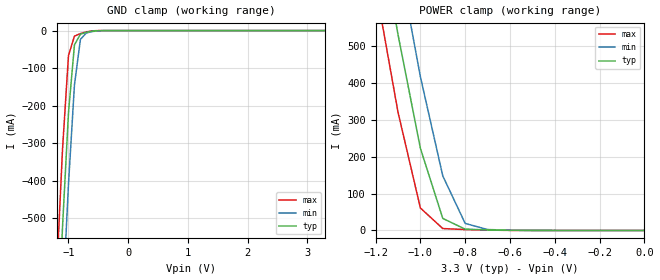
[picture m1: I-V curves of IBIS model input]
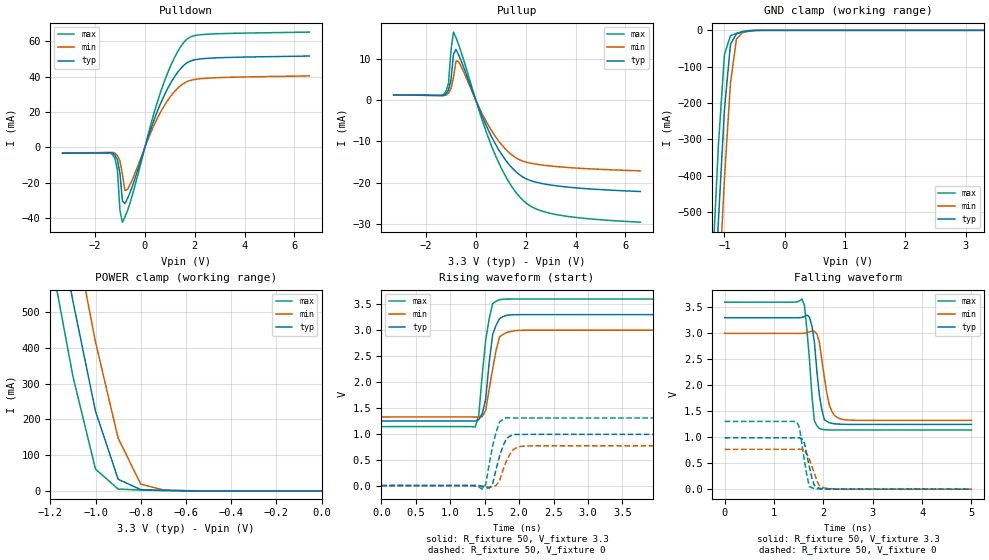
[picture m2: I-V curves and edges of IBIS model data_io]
| TSOP package & Industrial   Operation
[IBIS Ver]   3.2
[Comment Char]   |_char
[File name]   as7c31026b_tsopi.ibs
[File Rev]   1.0
[Date]   May 19, 2004 3:37:27 PM
[Source]
Alliance Semiconductor Corporation
[Notes]
This model  is for TSOP package &
 Industrial  Operation
[Disclaimer]
Data is for modeling purpose only and is not guaranted.
This IBIS model is provided on an "AS IS" basis and Alliance Semiconductor makes
absolutely no warranty with respect to the information contained
herein.The entire risk as to quality and performance
is with the Customer. ACCORDINGLY, IN NO EVENT SHALL THE COMPANY BE
LIABLE FOR ANY DAMAGES, WHETHER IN CONTRACT OR TORT,INCLUDING ANY
LOST PROFITS OR OTHER INCIDENTAL, CONSEQUENTIAL, EXEMPLARY, OR
PUNITIVE DAMAGES ARISING OUT OF THE USE OR APPLICATION OF THE IBIS
model provided in this package.
[Copyright]
Alliance Semiconductor Corporation
| tsop Package & Industrial Operation.
[Component]   AS7C31026B_TSOPI
Si_location Pin
Timing_location Pin
[Manufacturer]   Alliance Semiconductor Corporation
[Package]
R_pkg   321.15m   142.5m   499.8m
L_pkg   5.882nH   2.534nH   9.23nH
C_pkg   1.013pF   0.614pF   1.412pF
[Pin] signal_name   model_name
1   A4   input
2   A3   input
3   A2   input
4   A1   input
5   A0   input
6   NCE   input
7   IO0   data_io
8   IO1   data_io
9   IO2   data_io
10   IO3   data_io
11   VCC   POWER
12   GND   GND
13   IO4   data_io
14   IO5   data_io
15   IO6   data_io
16   IO7   data_io
17   NWE   input
18   A15   input
19   A14   input
20   A13   input
21   A12   input
22   NC   NC
23   NC   NC
24   A11   input
25   A10   input
26   A9   input
27   A8   input
28   NC   NC
29   IO8   data_io
30   IO9   data_io
31   IO10   data_io
32   IO11   data_io
33   VCC   POWER
34   GND   GND
35   IO12   data_io
36   IO13   data_io
37   IO14   data_io
38   IO15   data_io
39   NLB   input
40   NUB   input
41   NOE   input
42   A7   input
43   A6   input
44   A5   input
| Models and submodels in the file (2): input (Input), data_io (I/O)
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[Model]   input
Model_type Input
Vinh=2V
Vinl=0.8V
C_comp   4pF   4pF   4pF
[Model Spec]
[Temperature Range] 25   85   -40
[Voltage Range]   3.3   3.0   3.6
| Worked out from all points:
|   GND clamp passes 1 mA (typ) near -0.56 V on its own axis
|   POWER clamp passes 1 mA (typ) near -0.65 V on its own axis
[GND Clamp]
-3.3V     -8.605A    -8.704A    -8.517A
-1.2V     -871.8mA   -1.087A    -656.4mA
-1.1V     -525.3mA   -736.1mA   -317.8mA
-1V       -219.6mA   -410.1mA   -66.68mA
-900mV    -38.16mA   -145.2mA   -14.81mA
-800mV    -9.652mA   -23.43mA   -8.009mA
-700mV    -4.621mA   -6.209mA   -3.26mA
-600mV    -1.581mA   -2.49mA    -667.7uA
-300mV    -1.257uA   -9.648uA   -37.29nA
3.3V      156pA      2.475uA    72.11pA
[POWER Clamp]
-3.3V     8.613A     8.714A     8.524A
-1.2V     879.9mA    1.098A     661.8mA
-1.1V     531.7mA    745.4mA    321mA
-1V       222.9mA    417mA      61.01mA
-900mV    32.63mA    148mA      5.18mA
-800mV    3.618mA    19.12mA    2.468mA
-700mV    1.463mA    2.534mA    1.021mA
0V        156pA      3.437nA    86.52pA
[Model]   data_io
Model_type I/O
Enable Active-High
Polarity Non-Inverting
Vinh=2V
Vinl=0.8V
Vref=1.728V
Vmeas=1.5V
Rref=168
Cref=30pF
C_comp   4pF   4pF   4pF
[Temperature Range] 25   85   -40
[Voltage Range]   3.3   3.0   3.6
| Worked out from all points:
|   slope of the pulldown table from 0 to 0.495 V, typ, clamps not added: 24.6 ohm
|   slope of the pullup table from 0 to 0.495 V, typ, clamps not added: 68.8 ohm
|   GND clamp passes 1 mA (typ) near -0.56 V on its own axis
|   POWER clamp passes 1 mA (typ) near -0.65 V on its own axis
|   falling waveform, R_fixture 50, V_fixture 3.3: 20-80 % time 137ps typ, 169ps min, 123ps max; typ from 3.3 V to 1.25 V
|   falling waveform, R_fixture 50, V_fixture 0: 20-80 % time 138ps typ, 177ps min, 128ps max; typ from 0.987 V to 0.001 V
|   rising waveform, R_fixture 50, V_fixture 3.3: 20-80 % time 101ps typ, 136ps min, 120ps max; typ from 1.25 V to 3.3 V
|   rising waveform, R_fixture 50, V_fixture 0: 20-80 % time 131ps typ, 141ps min, 123ps max; typ from 0 V to 0.988 V
[Pullup]
-3.3V     1.309mA    1.306mA    1.287mA
-1.3V     1.177mA    1.138mA    1.428mA
-1.1V     2.464mA    1.747mA    4.103mA
-1V       4.894mA    2.775mA    12.12mA
-900mV    11.13mA    5.513mA    16.58mA
-800mV    12.37mA    9.544mA    15.24mA
-700mV    11.15mA    9.475mA    13.65mA
700mV     -9.696mA   -8.061mA   -12.18mA
1.2V      -14.6mA    -11.94mA   -18.57mA
1.8V      -18.3mA    -14.57mA   -23.75mA
3.1V      -20.68mA   -16.03mA   -27.62mA
6.6V      -22.17mA   -17.15mA   -29.63mA
[Pulldown]
-3.3V     -3.25mA    -3.127mA   -3.217mA
-1.3V     -3.123mA   -2.802mA   -3.951mA
-1.1V     -7.003mA   -4.598mA   -12.7mA
-1V       -14.54mA   -7.558mA   -35.58mA
-900mV    -30.21mA   -15.21mA   -42.2mA
-800mV    -31.71mA   -24.25mA   -39.29mA
-700mV    -28.96mA   -23.7mA    -35.77mA
600mV     23.78mA    19.12mA    29.92mA
1.1V      37.92mA    30.08mA    48.14mA
1.6V      46.83mA    36.54mA    59.97mA
2.4V      50.22mA    39.03mA    63.86mA
6.6V      51.64mA    40.41mA    65.16mA
[GND Clamp]
-3.3V     -8.605A    -8.704A    -8.517A
-1.2V     -871.8mA   -1.087A    -656.4mA
-1.1V     -525.3mA   -736.1mA   -317.8mA
-1V       -219.6mA   -410.1mA   -66.68mA
-900mV    -38.16mA   -145.2mA   -14.81mA
-800mV    -9.652mA   -23.43mA   -8.009mA
-700mV    -4.621mA   -6.209mA   -3.26mA
-600mV    -1.581mA   -2.49mA    -667.7uA
-300mV    -1.257uA   -9.648uA   -37.29nA
3.3V      156pA      2.475uA    72.11pA
[POWER Clamp]
-3.3V     8.613A     8.714A     8.524A
-1.2V     879.9mA    1.098A     661.8mA
-1.1V     531.7mA    745.4mA    321mA
-1V       222.9mA    417mA      61.01mA
-900mV    32.63mA    148mA      5.18mA
-800mV    3.618mA    19.12mA    2.468mA
-700mV    1.463mA    2.534mA    1.021mA
0V        156pA      3.437nA    86.52pA
[Falling Waveform]
R_fixture=50
V_fixture=3.3
V_fixture_min=3.0
V_fixture_max=3.6
0s        3.3V       3V         3.6V
1.566ns   3.307V     2.998V     3.658V
1.616ns   3.322V     3.002V     3.533V
1.768ns   3.14V      3.044V     1.798V
1.818ns   2.827V     3.037V     1.312V
1.919ns   1.806V     2.828V     1.165V
2.02ns    1.339V     2.147V     1.145V
2.121ns   1.279V     1.616V     1.141V
2.323ns   1.253V     1.362V     1.138V
5ns       1.247V     1.324V     1.138V
[Falling Waveform]
R_fixture=50
V_fixture=0
V_fixture_min=0
V_fixture_max=0
0s        987.1mV    766.3mV    1.303V
1.465ns   991.4mV    768.5mV    1.289V
1.515ns   988.3mV    769mV      1.184V
1.616ns   884.2mV    744.4mV    551.3mV
1.667ns   650.4mV    671.7mV    253.7mV
1.717ns   425.3mV    576.7mV    50.02mV
1.818ns   72.24mV    300.3mV    13.11mV
1.919ns   18.85mV    70.48mV    4.731mV
2.121ns   4.21mV     12.82mV    1.16mV
5ns       1.203mV    1.263mV    1.144mV
[Rising Waveform]
R_fixture=50
V_fixture=3.3
V_fixture_min=3.0
V_fixture_max=3.6
0s        1.246V     1.323V     1.137V
1.364ns   1.244V     1.323V     1.132V
1.414ns   1.273V     1.324V     1.347V
1.465ns   1.383V     1.33V      2.132V
1.515ns   1.672V     1.455V     2.805V
1.566ns   2.377V     1.859V     3.217V
1.616ns   2.915V     2.25V      3.511V
1.717ns   3.224V     2.871V     3.587V
2.02ns    3.298V     2.996V     3.598V
5ns       3.298V     2.998V     3.598V
[Rising Waveform]
R_fixture=50
V_fixture=0
V_fixture_min=0
V_fixture_max=0
0s        0V         0V         0V
1.313ns   1.468mV    1.422mV    -625.9uV
1.465ns   -22.26mV   -5.326mV   -68.63mV
1.515ns   -39.5mV    -14.66mV   19.86mV
1.616ns   36.55mV    -29.42mV   770.1mV
1.717ns   571.3mV    98.57mV    1.229V
1.818ns   909.9mV    482.6mV    1.31V
1.919ns   985.4mV    699.2mV    1.305V
2.071ns   987.8mV    761.6mV    1.304V
5ns       988.3mV    767.6mV    1.304V
[Ramp]
R_load=50
dV/dt_r   5.930E-1/1.286E-10   4.606E-1/1.404E-10   7.825E-1/1.220E-10
dV/dt_f   1.232E+0/1.330E-10   1.006E+0/1.599E-10   1.477E+0/1.179E-10
|[End   data_io
